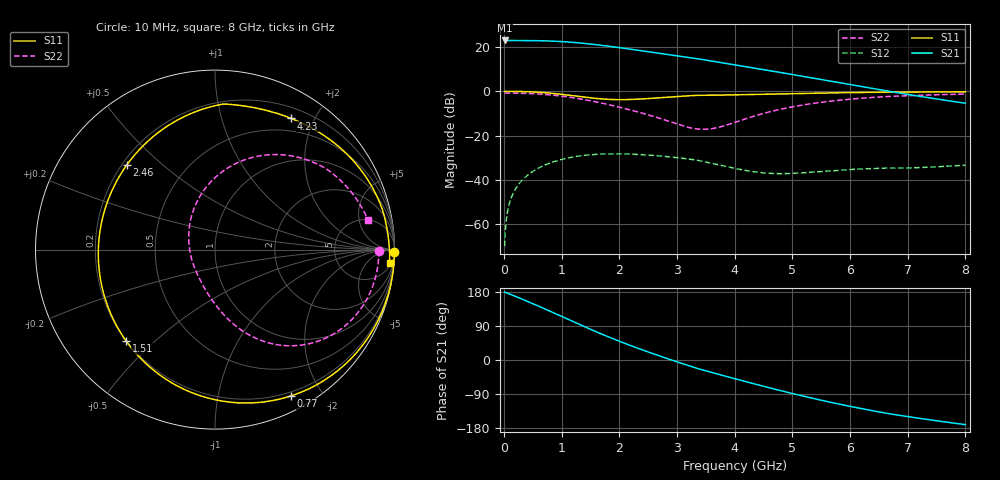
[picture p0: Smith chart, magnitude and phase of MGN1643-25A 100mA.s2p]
! Port[1] = GATE
! Port[2] = DRAIN
! [Type]  S-parameter s2p file touchstone ver. 1.0
! [Object]  MGN1643-25A
! [Bias]  100 mA
! [Version]  1.0
! [Date]  Tue May 19 13:03:48 2026
! [Source]  This file was created in JSC "ICC Milandr".
! [Disclaimer] Property of JSC "ICC Milandr". Unauthorized reproduction and/or distribution is strictly prohibited.
!  The file and the data are provided "AS IS" and with all faults and disclaim all warranties, express and implied, including
!  without limitation any implied warranties of merchantability, fitness for a particular purpose.
!  JSC "ICC Milandr" assumes no liability for:
!  1) the accuracy of the data provided;
!  2) the proper functioning of this data;
!  3) infringement of patents, copyrights or intellectual property rights resulting from the use of this data.
!  JSC "ICC Milandr" reserves the right to make changes to the products and the data without prior notice.
!  Please, be aware that your receipt and use of the file provided shall serve as acceptance of these terms and conditions.
!  If you do not accept these terms, you should return or destroy this file and any other accompanying information immediately.
# Hz S MA R 12.5
! freq  S11mag  S11ang  S21mag  S21ang  S12mag  S12ang  S22mag  S22ang
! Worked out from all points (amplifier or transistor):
!   800 points, 10 MHz to 8 GHz, reference 12.5 ohm
!   highest |S21| = 23.0 dB at 10 MHz (marker M1)
!   |S21| within 3 dB of that: start of sweep to 1.931 GHz
!   unconditionally stable (mu >= 1): 2.813 GHz to 7.008 GHz
!   at 1.34 GHz: K = 0.47, MSG = 25.4 dB, |S12| = -29.1 dB
!   at 4.01 GHz: K = 1.93, MAG = 17.8 dB, |S12| = -34.8 dB
!   at 8 GHz: K = 0.63, MSG = 14.0 dB, |S12| = -33.4 dB
!   S11 on the Smith chart (normalised r, x): 10 MHz: open; 770 MHz: 0.16, -1.63; 1.51 GHz: 0.20, -0.41; 2.46 GHz: 0.22, +0.39; 4.23 GHz: 0.33, +1.69; 8 GHz: 8, -24
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1e7  0.9998 -0.7  14.1 179.2  0.000318 82.6  0.9134 -0.4
1.3e8  0.9987 -10.0  14.07 172.1  0.004084 82.5  0.9121 -5.1
3.9e8  0.983 -30.6  14.03 155.8  0.01219 68.3  0.8967 -15.4
5.8e8  0.9572 -46.2  13.93 143.3  0.01792 57.3  0.8729 -23.2
7.7e8  0.9184 -62.6  13.73 130.5  0.02329 46.0  0.8371 -30.9
1.06e9  0.8387 -89.2  13.15 110.7  0.03027 28.3  0.7607 -42.6
1.2e9  0.7961 -102.8  12.76 101.0  0.03294 19.8  0.7161 -48.0
1.35e9  0.7517 -117.9  12.26 90.9  0.03523 10.8  0.6647 -53.6
1.51e9  0.71 -134.3  11.67 80.2  0.03701 1.4  0.6079 -59.3
1.74e9  0.6673 -158.3  10.76 65.4  0.03844 -11.5  0.5263 -66.9
1.96e9  0.6498 179.4  9.868 51.9  0.03874 -23.3  0.4519 -73.7
2.2e9  0.6551 157.1  8.933 37.8  0.03812 -35.3  0.3773 -81.1
2.46e9  0.6813 136.0  7.996 23.3  0.03663 -47.6  0.3048 -89.8
2.68e9  0.7126 120.8  7.276 11.6  0.03488 -57.5  0.2501 -98.9
3e9  0.7625 102.4  6.349 -4.9  0.03177 -71.2  0.1829 -118.4
3.32e9  0.81 87.4  5.547 -20.8  0.02817 -84.3  0.1431 -152.0
4.01e9  0.8336 65.6  3.94 -49.7  0.01814 -87.4  0.2006 134.4
4.23e9  0.8452 59.9  3.536 -58.6  0.01602 -84.2  0.2495 119.0
4.78e9  0.8769 47.1  2.685 -80.2  0.01382 -70.4  0.3901 91.7
5.34e9  0.9075 35.9  2.011 -100.6  0.01495 -60.7  0.5293 71.4
6.67e9  0.9591 13.6  1.005 -141.6  0.01846 -64.2  0.7662 36.0
8e9  0.9756 -4.3  0.5382 -170.6  0.02142 -85.1  0.8679 11.1
